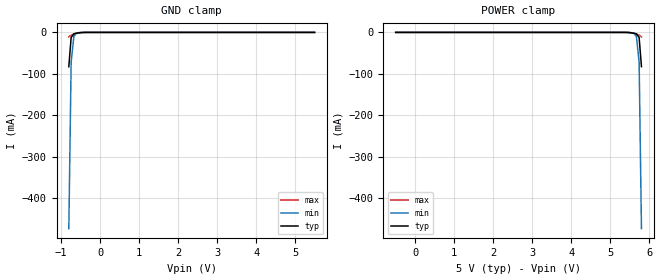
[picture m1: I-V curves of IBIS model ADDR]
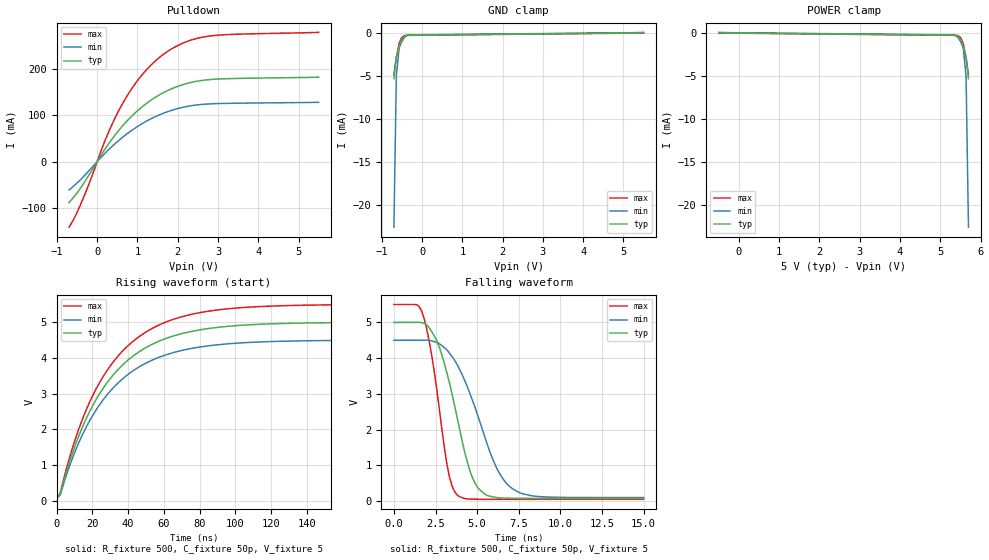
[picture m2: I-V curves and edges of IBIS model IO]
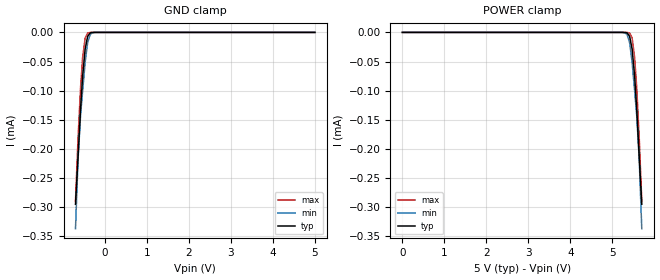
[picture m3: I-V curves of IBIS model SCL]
[IBIS Ver]   3.2
[Comment Char]   |_char
| VDD nom = 5v, min = 4.5v, max =5.5v
[File name]   pca8575_5v.ibs
[File Rev]   1
[Date]   Aug 14, 2008 2:49:03 PM
[Source]
Generated by Seshadri Venkataramanan using IBIS Toolkit at NXP Tempe
[Notes]
[Disclaimer]
(C) Copyright 2007 NXP Semiconductors
All rights reserved
NXP Semiconductors (NXP) does not warrant that this model and any other
accompanying information (Model) accurately or fully represents the
operating characteristics and specifications of the semiconductor
products to which the Model relates.  Moreover, the Model is furnished
on an "as is" and with "all faults" basis, and without support or
warranty of any kind.  NXP disclaims all warranties, whether expressed
or implied or statutory, including without limitation all implied
warranties of non-infringement, merchantability and fitness for any
purpose, and those arising from a course of dealing or usage of trade.
NXP does not convey any license under its or any third party's patents,
copyrights or other intellectual property or proprietary rights.
You and your company assume any and all risks and liability arising out
of the application or use of the Model.
In no event shall NXP be liable for any direct, indirect, special,
consequential or incidental damages, however caused, whether in
warranty, contract or tort (including negligence), strict liability or
other legal theory, including, without limitation, for lost profits,
business interruption, or corruption or loss of data or information,
arising out of or in connection with the use of or the inability to use
the Model, even if NXP has been advised of the possibility of such
damages.
NXP provides the Model as a courtesy to our customers. You and your
company shall not distribute, convey, sell, or give the Model to anyone
else without receiving prior written permission from NXP.
NXP reserves the right to make changes without notice to the Model to
improve reliability, function, or design.
Please be aware that your receipt and subsequent use of the Model shall
serve as acceptance of these terms and conditions.  If you do not
accept these terms, return or destroy the Model immediately.
[Copyright]
2008
| SO24 package
[Component]   PCA8575D
Si_location Pin
Timing_location Pin
[Manufacturer]   NXP Semiconductors
[Package]
R_pkg   0.14   0.12   0.18
L_pkg   5.71n   3.95n   7.95n
C_pkg   1.01p   0.72p   1.49p
[Pin] signal_name   model_name   R_pin   L_pin   C_pin
1   INTb   INT_OUT   0.18   6.01n   0.97p
2   AD1   ADDR   0.14   7.94n   1.21p
3   AD2   ADDR   0.16   7.06n   1.32p
4   P00   IO   0.18   6.01n   1.07p
5   P01   IO   0.14   4.98n   0.88p
6   P02   IO   0.13   4.30n   0.80p
7   P03   IO   0.12   3.95n   0.74p
8   P04   IO   0.12   3.95n   0.72p
9   P05   IO   0.13   4.30n   0.76p
10   P06   IO   0.14   4.98n   0.85p
11   P07   IO   0.18   6.01n   0.97p
12   VSS   GND   0.16   7.06n   1.20p
13   P10   IO   0.14   7.95n   1.45p
14   P11   IO   0.14   7.95n   1.49p
15   P12   IO   0.16   7.06n   1.32p
16   P13   IO   0.18   6.01n   1.07p
17   P14   IO   0.14   4.98n   0.88p
18   P15   IO   0.13   4.30n   0.80p
19   P16   IO   0.12   3.95n   0.74p
20   P17   IO   0.12   3.95n   0.72p
21   AD0   ADDR   0.13   4.30n   0.76p
22   SCL   SCL   0.14   4.98n   0.85p
23   SDA   SDAIO   0.18   6.01n   0.97p
24   VDD   POWER   0.16   7.06n   1.20p
| TSSOP24 package
[Component]   PCA8575PW
Si_location Pin
Timing_location Pin
[Manufacturer]   NXP Semiconductors
[Package]
R_pkg   52.70m   31.50m   67.00m
L_pkg   2.19n   1.32n   3.39n
C_pkg   0.48p   0.35p   0.93p
[Pin] signal_name   model_name   R_pin   L_pin   C_pin
1   INTb   INT_OUT   66.40m   2.36n   0.47p
2   AD1   ADDR   66.10m   3.39n   0.57p
3   AD2   ADDR   67.00m   2.94n   0.59p
4   P00   IO   66.40m   2.36n   0.47p
5   P01   IO   47.10m   1.67n   0.40p
6   P02   IO   38.00m   1.44n   0.37p
7   P03   IO   31.50m   1.32n   0.35p
8   P04   IO   31.50m   1.32n   0.35p
9   P05   IO   38.00m   1.44n   0.37p
10   P06   IO   47.10m   1.67n   0.40p
11   P07   IO   66.40m   2.36n   0.47p
12   VSS   GND   67.00m   2.94n   0.59p
13   P10   IO   66.10m   3.39n   0.61p
14   P11   IO   66.20m   3.39n   0.61p
15   P12   IO   67.00m   2.94n   0.59p
16   P13   IO   66.50m   2.36n   0.47p
17   P14   IO   47.10m   1.67n   0.40p
18   P15   IO   38.00m   1.45n   0.37p
19   P16   IO   31.50m   1.32n   0.35p
20   P17   IO   31.50m   1.32n   0.35p
21   AD0   ADDR   38.00m   1.45n   0.37p
22   SCL   SCL   47.10m   1.67n   0.40p
23   SDA   SDAIO   66.50m   2.36n   0.47p
24   VDD   POWER   67.00m   2.94n   0.59p
| SSOP24
[Component]   PCA8575DB
Si_location Pin
Timing_location Pin
[Manufacturer]   NXP Semiconductors
[Package]
R_pkg   54.20m   39.70m   64.80m
L_pkg   2.55n   1.89n   3.58n
C_pkg   0.636p   0.52p   1.05p
[Pin] signal_name   model_name   R_pin   L_pin   C_pin
1   INTb   INT_OUT   63.00m   2.53n   0.58p
2   AD1   ADDR   61.20m   3.56n   0.70p
3   AD2   ADDR   64.80m   3.10n   0.76p
4   P00   IO   63.00m   2.53n   0.60p
5   P01   IO   52.60m   2.17n   0.57p
6   P02   IO   43.90m   2.03n   0.56p
7   P03   IO   39.70m   1.89n   0.54p
8   P04   IO   39.70m   1.89n   0.52p
9   P05   IO   43.90m   2.03n   0.55p
10   P06   IO   52.60m   2.17n   0.56p
11   P07   IO   63.00m   2.53n   0.58p
12   VSS   GND   64.80m   3.10n   0.71p
13   P10   IO   61.20m   3.56n   1.01p
14   P11   IO   61.20m   3.56n   1.05p
15   P12   IO   64.80m   3.10n   0.80p
16   P13   IO   63.00m   2.53n   0.65p
17   P14   IO   52.60m   2.17n   0.59p
18   P15   IO   43.90m   2.03n   0.56p
19   P16   IO   39.70m   1.89n   0.54p
20   P17   IO   39.70m   1.89n   0.53p
21   AD0   ADDR   43.90m   2.03n   0.56p
22   SCL   SCL   52.60m   2.17n   0.57p
23   SDA   SDAIO   63.00m   2.53n   0.60p
24   VDD   POWER   64.80m   3.10n   0.76p
[Define Package Model]  HVQFN24
[Manufacturer]  ST-NXP Wireless
|[Simulated] Chris Hunat
|[Approved] Wayne Nunn, Roger Real
[OEM]  Unknown
[Description]  Full package model
[Number Of Pins]  23
[Pin Numbers]
pin1   | pin1 = lead1
pin2   | pin2 = lead2
pin3   | pin3 = lead3
pin4   | pin4 = lead4
pin5   | pin5 = lead5
pin6   | pin6 = lead6
pin7   | pin7 = lead7
pin8   | pin8 = lead8
pin9   | pin9 = lead9
pin10   | pin10 = lead10
pin11   | pin11 = lead11
pin12   | pin12 = lead12
pin13   | pin13 = lead13
pin14   | pin14 = lead14
pin15   | pin15 = lead15
pin17   | pin17 = lead17
pin18   | pin18 = lead18
pin19   | pin19 = lead19
pin20   | pin20 = lead20
pin21   | pin21 = lead21
pin22   | pin22 = lead22
pin23   | pin23 = lead23
pin24   | pin24 = lead24
[Model Data]
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[End Model Data]
[End Package Model]
[Define Package Model]  DHVQFN24
[Manufacturer]  ST-NXP Wireless
|[Simulated] Chris Hunat
|[Approved] Wayne Nunn, Roger Real
[OEM]  Unknown
[Description]  Full package model
[Number Of Pins]  24
[Pin Numbers]
|Pin Num   Terminal Name
1   | lead1:pin1
2   | lead2:pin2
3   | lead3:pin3
4   | lead4:pin4
5   | lead5:pin5
6   | lead6:pin6
7   | lead7:pin7
8   | lead8:pin8
9   | lead9:pin9
10   | lead10:pin10
11   | lead11:pin11
12   | lead12:pin12
13   | lead13:pin13
14   | lead14:pin14
15   | lead15:pin15
16   | lead16:pin16
17   | lead17:pin17
18   | lead18:pin18
19   | lead19:pin19
20   | lead20:pin20
21   | lead21:pin21
22   | lead22:pin22
23   | lead23:pin23
24   | lead24:pin24
[Model Data]
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[End Model Data]
[End Package Model]
| Models and submodels in the file (5): ADDR (Input), IO (I/O_open_drain), SCL (Input), SDAIO (I/O_open_drain), INT_OUT (Open_drain)
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[Model]   ADDR
Model_type Input
Vinh=3.5
Vinl=1.5
C_comp   0.73p   0.7p   0.76p
[Temperature Range] 27   85   -40
[Voltage Range]   5   4.5   5.5
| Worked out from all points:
|   GND clamp passes 1 mA (typ) near -0.54 V on its own axis
[GND Clamp]
-800mV    -82.74mA   -473.3mA   -10.75mA
-740mV    -12.18mA   -71.08mA   -6.58mA
-670mV    -3.609mA   -9.611mA   -3.955mA
-610mV    -2.203mA   -2.754mA   -1.946mA
-290mV    -1.019uA   -5.279uA   -58.36nA
5.5V      106.9pA    399pA      72.28pA
[POWER Clamp]
-500mV    106.9pA    399pA      72.28pA
5.29V     -1.019uA   -5.279uA   -58.36nA
5.61V     -2.203mA   -2.754mA   -1.946mA
5.67V     -3.609mA   -9.611mA   -3.955mA
5.74V     -12.18mA   -71.08mA   -6.58mA
5.8V      -82.74mA   -473.3mA   -10.75mA
[Model]   IO
Model_type I/O_open_drain
Vinh=3.5
Vinl=1.5
Vref=5
Vmeas=2.5
Rref=500
Cref=50p
C_comp   6.3p   6.1p   6.5p
[Temperature Range] 27   85   -40
[Voltage Range]   5   4.5   5.5
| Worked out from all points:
|   slope of the pulldown table from 0 to 0.75 V, typ, clamps not added: 8.51 ohm
|   GND clamp passes 1 mA (typ) near -0.52 V on its own axis
|   falling waveform, R_fixture 500, C_fixture 50p, V_fixture 5: 20-80 % time 1.51ns typ, 2.11ns min, 1.01ns max; typ from 5 V to 0.069 V
|   rising waveform, R_fixture 500, C_fixture 50p, V_fixture 5: 20-80 % time 34.7ns typ, 34.8ns min, 34.6ns max; typ from 0.069 V to 5 V
[Pulldown]
-700mV    -87.8mA    -60.93mA   -140.7mA
-570mV    -74.83mA   -51.24mA   -121.6mA
-390mV    -53.69mA   -36.64mA   -87.54mA
240mV     32.93mA    22.02mA    54.81mA
550mV     68.73mA    46.63mA    112.1mA
800mV     92.82mA    63.63mA    149.3mA
1.05V     113.1mA    78.24mA    179.7mA
1.3V      130mA      90.57mA    204.3mA
1.62V     147.1mA    103.3mA    228.9mA
2.12V     165.3mA    116.6mA    254.3mA
2.74V     175.9mA    123.8mA    269.3mA
5.5V      181.5mA    127.5mA    277.8mA
[GND Clamp]
-700mV    -5.295mA   -22.53mA   -4.852mA
-640mV    -2.786mA   -4.999mA   -2.841mA
-570mV    -1.638mA   -1.736mA   -1.224mA
-510mV    -829.9uA   -1.059mA   -553.2uA
-450mV    -423.5uA   -584.2uA   -325uA
-390mV    -281.8uA   -320.2uA   -280.9uA
-200mV    -239.8uA   -212.7uA   -267.2uA
5.5V      23.22uA    77.99uA    169.3pA
[POWER Clamp]
-500mV    23.22uA    77.99uA    169.3pA
5.2V      -239.8uA   -212.7uA   -267.2uA
5.39V     -281.8uA   -320.2uA   -280.9uA
5.45V     -423.5uA   -584.2uA   -325uA
5.51V     -829.9uA   -1.059mA   -553.2uA
5.57V     -1.638mA   -1.736mA   -1.224mA
5.64V     -2.786mA   -4.999mA   -2.841mA
5.7V      -5.295mA   -22.53mA   -4.852mA
[Falling Waveform]
R_fixture=500
C_fixture=50p
V_fixture=5
V_fixture_min=4.5
V_fixture_max=5.5
0s        5V         4.5V       5.5V
1.364ns   5.001V     4.5V       5.495V
1.818ns   4.976V     4.502V     5.106V
2.273ns   4.736V     4.483V     4.072V
3.182ns   3.589V     4.233V     1.04V
3.788ns   2.362V     3.83V      170.6mV
5ns       399.5mV    2.443V     47.2mV
6.212ns   91.66mV    883.3mV    45.28mV
7.121ns   73.85mV    343.8mV    44.96mV
15ns      69.04mV    94.26mV    44.8mV
[Rising Waveform]
R_fixture=500
C_fixture=50p
V_fixture=5
V_fixture_min=4.5
V_fixture_max=5.5
0s        69.03mV    93.83mV    44.8mV
2.02ns    185.6mV    161.2mV    215.8mV
6.061ns   899.4mV    801.7mV    1.002V
12.12ns   1.779V     1.593V     1.97V
24.24ns   3.014V     2.705V     3.328V
36.36ns   3.777V     3.393V     4.165V
52.53ns   4.36V      3.919V     4.802V
70.71ns   4.691V     4.219V     5.164V
96.97ns   4.892V     4.402V     5.383V
200ns     4.998V     4.498V     5.498V
[Ramp]
R_load=500
dV/dt_r   2.959E+0/8.796E-10   2.931E+0/9.723E-10   2.982E+0/7.822E-10
dV/dt_f   2.959E+0/3.531E-10   2.930E+0/6.173E-10   2.982E+0/2.018E-10
|[End   IO
[Model]   SCL
Model_type Input
Vinh=3.5
Vinl=1.5
C_comp   2.1p   1.9p   2.3p
[Temperature Range] 27   85   -40
[Voltage Range]   5   4.5   5.5
[GND Clamp]
-700mV    -295uA     -337uA     -289.5uA
-640mV    -215uA     -219.5uA   -182.9uA
-580mV    -132.2uA   -142.9uA   -95.46uA
-530mV    -75.1uA    -100.5uA   -43.1uA
-470mV    -28.59uA   -51.28uA   -9.682uA
-410mV    -6.63uA    -17.35uA   -1.079uA
-350mV    -920.5nA   -3.647uA   -77.68nA
-300mV    -138.4nA   -722.3nA   -7.551nA
-180mV    -1.06nA    -8.721nA   -23.84pA
5V        12pA       33.5pA     10.02pA
[POWER Clamp]
0V        12pA       33.5pA     10.02pA
5.18V     -1.06nA    -8.721nA   -23.84pA
5.3V      -138.4nA   -722.3nA   -7.551nA
5.35V     -920.5nA   -3.647uA   -77.68nA
5.41V     -6.63uA    -17.35uA   -1.079uA
5.47V     -28.59uA   -51.28uA   -9.682uA
5.53V     -75.1uA    -100.5uA   -43.1uA
5.58V     -132.2uA   -142.9uA   -95.46uA
5.64V     -215uA     -219.5uA   -182.9uA
5.7V      -295uA     -337uA     -289.5uA
